FUNCTION_BLOCK "IMAC_MOTOR1"
TITLE = MOTOR 1
//--------------------------------------------------------------------------------
//SIEMENS AG     I&S IP PEP SN                       PSP-Element: D-09300081-E-E5
//--------------------------------------------------------------------------------
//History
//=======
//Date      Version  Description                        Author
//1997/06/09   0.6   Basic Edition                      Salge
//2004/06/02   1.0   Converted to S7                    Kahle
//2004/11/29   1.1   Anypointer adjusted                Edelmann
//2004/12/07   1.2   Interface adapted                  Edelmann
//
//--------------------------------------------------------------------------------
//PLC:   >= S7-300
//--------------------------------------------------------------------------------
//Specification:   Refer "TECHFUNK.DOC"
//--------------------------------------------------------------------------------
//
//--------------------------------------------------------------------------------
//Called FC: FC90 "DELAYTIMER"
//           SFC20 "BLKMOV"
//--------------------------------------------------------------------------------
//
//--------------------------------------------------------------------------------
//Note:
//--------------------------------------------------------------------------------
// KNOW_HOW_PROTECT
AUTHOR : Sa_Ka
FAMILY : IMAC
NAME : Motor1
VERSION : 1.2


VAR_INPUT
  OBJ : INT ;	//current used object
  RMOT : BOOL ;	//mode remote (=1) is activated
  RUN : BOOL ;	//Feedback Motor is running
  FAUL : BOOL ;	//Feedback Motor fault
  BLKO : BOOL ;	//Blackout indication
  ACOM : WORD ;	//Automatic commands
  PCONF : STRUCT
   LastRecord : INT  := 100;
   Pointer1stRecord : STRUCT
    S7ID : BYTE  := B#16#10;	//ANY pointer: ID S7
    Typ : BYTE  := B#16#2;	//ANY pointer: data typ =02 BYTE =04 WORD =05 INT =06 DWORD =07 DINT =08 REAL
    RepeatFactor : INT  := 104;	//ANY pointer: repeat factor
    DBNo : INT  := 80;	//ANY pointer: DB number, zero if no DB
    MemoryArea : BYTE  := B#16#84;	//ANY pointer: Memory area =81 IN =82 OUT =83 M =84 DB =85 DI =86 L
    DWHigh : BYTE ;	//ANY pointer: DW highest byte
    DWX : INT ;	//ANY pointer: DW low / bit (address = byte *8 + bit)
   END_STRUCT ;
  END_STRUCT ;
END_VAR
VAR_OUTPUT
  MSTA : BOOL ;	//Command Start Motor
  MSTO : BOOL ;	//Command Stop Motor
  ASTAT : WORD ;	//Status as feedback for the automatic
//******************** CODE SECTION ********
  OSSTAT : WORD ;	//Status for OS
  OSALARM : WORD ;	//Alarms for OS
END_VAR
VAR_IN_OUT
  OSCOM : WORD ;
END_VAR
VAR
  Motor1 : STRUCT
   System : WORD ;
   CmdOS : WORD ;
   MirrorCmdOS : WORD ;
   Test : WORD ;
   AlarmOS : WORD ;
   StatusOS : WORD ;
   SysStatusOS : WORD ;
   Status1 : WORD ;
   Status2 : WORD ;
   InputEdges : WORD ;
   AutoEdges : WORD ;
   DataTimeCmd : STRUCT
    StartTime : DINT ;
    StartEdge : BOOL ;
   END_STRUCT ;
   DataTimeBlackout : STRUCT
    StartTime : DINT ;
    StartEdge : BOOL ;
   END_STRUCT ;
   DataTimeExtFault : STRUCT
    StartTime : DINT ;
    StartEdge : BOOL ;
   END_STRUCT ;
   DataTimeFeedback : STRUCT
    StartTime : DINT ;
    StartEdge : BOOL ;
   END_STRUCT ;
   DataTimeStrtActFault : STRUCT
    StartTime : DINT ;
    StartEdge : BOOL ;
   END_STRUCT ;
   DataTimeAutoAl : STRUCT
    StartTime : DINT ;
    StartEdge : BOOL ;
   END_STRUCT ;
   DataTimeRestart : STRUCT
    StartTime : DINT ;
    StartEdge : BOOL ;
   END_STRUCT ;
   DataTimeStpActFault : STRUCT
    StartTime : DINT ;
    StartEdge : BOOL ;
   END_STRUCT ;
   PCONF : STRUCT
    Modeswitches : STRUCT
     DlyAFaultStop : BOOL ;	//    Modeswitch Delayed Auto Fault with Stop
     sw01 : BOOL ;	//
     ExtFaultNC : BOOL ;	//    Modeswitch External fault NC
     sw03 : BOOL ;	//
     sw04 : BOOL ;	//
     sw05 : BOOL ;	//
     sw06 : BOOL ;	//
     sw07 : BOOL ;	//
     ConstOutput : BOOL ;	//    Modeswitch Constant Output
     ExtraAutomode : BOOL ;	//    Extra Automode
     NoActAFeedbackA : BOOL ;	//    Modeswitch No action and feedback alarm
     StopIfA : BOOL ;	//    Modeswitch Stop if alarm
     RestrtAftBlack : BOOL ;	//    Modeswitch Restart after Blackout
     RstAStartStop : BOOL ;	//    Modeswitch Reset Alarm with Start /Stop
     CmdTdly : BOOL ;	//    Modeswitch Command time delay
     LockBlockCmd : BOOL ;	//    Modeswitch Lock blocksCommands
    END_STRUCT ;
    DlyTCmd : TIME ;	// Setpoint command time delay
    DlyTBlackout : TIME ;	// Setpoint blackout time delay
    DlyTExtFault : TIME ;	// Setpoint external fault delay
    DlyTFeedback : TIME ;	// Setpoint feedback fault delay
    DlyTStrtActFault : TIME ;	//Setpoint start action delay
    DlyTAutoAl : TIME ;	// Setpoint auto alarm delay
    DlyTRestart : TIME ;	// Setpoint restart after blackout delay
    DlyTStpActFault : TIME ;	// Setpoint stop action fault
   END_STRUCT ;
  END_STRUCT ;
  siFailRR : INT ;	//Failure blockmove read record
  siFailWR : INT ;	//Failure blockmove write record
END_VAR
VAR_TEMP
  tb200_0 : BOOL ;	//
  tbCmdOSManual : BOOL ;	//    Command Manual
  tbCmdOSAuto : BOOL ;	//    Command Auto
  tb200_3 : BOOL ;	//
  tb200_4 : BOOL ;	//
  tb200_5 : BOOL ;	//
  tb200_6 : BOOL ;	//
  tb200_7 : BOOL ;	//
  tbCmdOSStart : BOOL ;	//    Command Start OS pulse
  tbCmdOSStop : BOOL ;	//    Command Stop OS pulse
  tb201_2 : BOOL ;	//
  tb201_3 : BOOL ;	//
  tb201_4 : BOOL ;	//
  tb201_5 : BOOL ;	//
  tb201_6 : BOOL ;	//
  tbCmdOSReset : BOOL ;	//    Command Reset OS pulse
  tbAutoBlackStart : BOOL ;	//    Blackoutstart from Auto
  tbAutoStbyCtrl : BOOL ;	//    Standbycontrol active
  tb202_2 : BOOL ;	//
  tb202_3 : BOOL ;	//
  tb202_4 : BOOL ;	//
  tb202_5 : BOOL ;	//
  tb202_6 : BOOL ;	//
  tbDataReq : BOOL ;	//    Fetch Data requiered
  tbAutoStart : BOOL ;	//
  tbAutoStop : BOOL ;	//
  tbAutoFail : BOOL ;	//    Auto failure input
  tbCmdLock : BOOL ;	//    Command Lock
  tbCmdEmergOff : BOOL ;	//    Command Emergency Off
  tb203_5 : BOOL ;	//
  tb203_6 : BOOL ;	//
  tb203_7 : BOOL ;	//
  tb204_0 : BOOL ;	//
  tb204_1 : BOOL ;	//
  tb204_2 : BOOL ;	//
  tb204_3 : BOOL ;	//
  tb204_4 : BOOL ;	//
  tb204_5 : BOOL ;	//
  tb204_6 : BOOL ;	//
  tb204_7 : BOOL ;	//
  tbCmdAutoStart : BOOL ;	//    Command Start Auto Pulse
  tbCmdAutoStop : BOOL ;	//    Command Stop Auto Pulse
  tbCmdAutoFail : BOOL ;	//    Auto failure input pulse
  tb205_3 : BOOL ;	//
  tb205_4 : BOOL ;	//
  tb205_5 : BOOL ;	//
  tb205_6 : BOOL ;	//
  tb205_7 : BOOL ;	//
  tbRemote : BOOL ;	//    Remote (=1)/ Local
  tbRunning : BOOL ;	//    Running (=1)/ Stopped
  tbFault : BOOL ;	//    Fault
  tbBlackout : BOOL ;	//    Blackout
  tb206_4 : BOOL ;	//
  tb206_5 : BOOL ;	//
  tb206_6 : BOOL ;	//
  tb206_7 : BOOL ;	//
  tb207_0 : BOOL ;	//
  tb207_1 : BOOL ;	//
  tb207_2 : BOOL ;	//
  tb207_3 : BOOL ;	//
  tb207_4 : BOOL ;	//
  tb207_5 : BOOL ;	//
  tb207_6 : BOOL ;	//
  tb207_7 : BOOL ;	//
  tb208_0 : BOOL ;	//
  tb208_1 : BOOL ;	//
  tb208_2 : BOOL ;	//
  tb208_3 : BOOL ;	//
  tb208_4 : BOOL ;	//
  tb208_5 : BOOL ;	//
  tb208_6 : BOOL ;	//
  tbSendData : BOOL ;	//    Send Data
  tbStateRun : BOOL ;	//    State Running
  tbStateLocal : BOOL ;	//    State Local
  tbStateManual : BOOL ;	//    State Manual
  tbStateAuto : BOOL ;	//    State Auto
  tbStateFault : BOOL ;	//    State Fault
  tbStateBlackout : BOOL ;	//    State Blackout
  tbStarting : BOOL ;	//    Starting
  tbReStarting : BOOL ;	//    ReStarting
  tb210_0 : BOOL ;
  tb210_1 : BOOL ;
  tb210_2 : BOOL ;
  tb210_3 : BOOL ;
  tb210_4 : BOOL ;
  tb210_5 : BOOL ;
  tb210_6 : BOOL ;
  tb210_7 : BOOL ;
  tb211_0 : BOOL ;
  tb211_1 : BOOL ;
  tb211_2 : BOOL ;
  tb211_3 : BOOL ;
  tb211_4 : BOOL ;
  tb211_5 : BOOL ;
  tb211_6 : BOOL ;
  tb211_7 : BOOL ;
  tb212_0 : BOOL ;
  tb212_1 : BOOL ;
  tb212_2 : BOOL ;
  tb212_3 : BOOL ;
  tb212_4 : BOOL ;
  tb212_5 : BOOL ;
  tb212_6 : BOOL ;
  tb212_7 : BOOL ;
  tb213_0 : BOOL ;
  tb213_1 : BOOL ;
  tb213_2 : BOOL ;
  tb213_3 : BOOL ;
  tb213_4 : BOOL ;
  tb213_5 : BOOL ;
  tb213_6 : BOOL ;
  tb213_7 : BOOL ;
  tbNonFeedbackTact : BOOL ;	//    Non Feedback Timer active
  tbNonFeedbackA : BOOL ;	//    Non Feedback Alarm
  tbStartTact : BOOL ;	//    Start Timer active
  tbActionA : BOOL ;	//    Action Alarm
  tbAutoTact : BOOL ;	//    Auto Timer active
  tbAutoA : BOOL ;	//    Auto Alarm
  tbRunBeforeBlack : BOOL ;	//    Running before blackout
  tbBlackoutStartTact : BOOL ;	//    Blackout start timer active
  tbStart : BOOL ;	//    Start
  tbStop : BOOL ;	//    Stop
  tbLocal : BOOL ;	//    Local
  tbManual : BOOL ;	//    Manual
  tbAuto : BOOL ;	//    Auto
  tbCmdTact : BOOL ;	//    Command Timer activ
  tbFaultTact : BOOL ;	//    Fault timer active
  tbExtFaultA : BOOL ;	//    Fault input alarm / external fault alarm
  tbMSTA : BOOL ;	//    Output MSTA
  tbMSTO : BOOL ;	//    Output MSTO
  tb216_2 : BOOL ;	//
  tb216_3 : BOOL ;	//
  tb216_4 : BOOL ;	//
  tb216_5 : BOOL ;	//
  tb216_6 : BOOL ;	//
  tb216_7 : BOOL ;	//
  tbDlyStop : BOOL ;	//    Delayed stop
  tbDlyStart : BOOL ;	//    Delayed start
  tbStopTact : BOOL ;	//    Stop Timer active
  tb217_3 : BOOL ;	//
  tb217_4 : BOOL ;	//
  tb217_5 : BOOL ;	//
  tb217_6 : BOOL ;	//
  tb217_7 : BOOL ;	//
  tbLtRpulse : BOOL ;	//    Local to remote pulse
  tb218_1 : BOOL ;	//
  tb218_2 : BOOL ;	//
  tb218_3 : BOOL ;	//
  tb218_4 : BOOL ;	//
  tb218_5 : BOOL ;	//
  tb218_6 : BOOL ;	//
  tb218_7 : BOOL ;	//
  tb219_0 : BOOL ;	//
  tb219_1 : BOOL ;	//
  tb219_2 : BOOL ;	//
  tb219_3 : BOOL ;	//
  tb219_4 : BOOL ;	//
  tb219_5 : BOOL ;	//
  tb219_6 : BOOL ;	//
  tb219_7 : BOOL ;	//
  tbCmdTexceed : BOOL ;	//Commnd delay time exceeded
  tbStartTexceed : BOOL ;	//Start delay time exceeded
  tbExtFTexceed : BOOL ;	//External fault delay time exceeded
  tbFeedbackTexceed : BOOL ;	//Feedback delay time exceeded
  tbAutoTexceed : BOOL ;	//Auto delay time exceeded
  tbBOStartTexceed : BOOL ;	//Blackout start delay time exceeded
  tb250_6 : BOOL ;
  tbStopTexceed : BOOL ;	//Stop delay time exceeded
  tbStartPulse : BOOL ;
  tbStopPulse : BOOL ;
  P_currentRecord : ANY ;	//ANY pointer of the current record
END_VAR
BEGIN
NETWORK
TITLE =Calculation of current ANY pointer for reading /writing record
// ANY-pointer of current record
      L     #PCONF.Pointer1stRecord.S7ID;
      T     LB    22;
      L     #PCONF.Pointer1stRecord.Typ;
      T     LB    23;
      L     #PCONF.Pointer1stRecord.RepeatFactor;
      T     LW    24;
      L     #PCONF.Pointer1stRecord.DBNo;
      T     LW    26;
      L     #PCONF.Pointer1stRecord.MemoryArea;
      T     LB    28;
      L     #PCONF.Pointer1stRecord.DWHigh;
      T     LB    29;
      L     #PCONF.Pointer1stRecord.DWX;
      T     LW    30;

      L     #OBJ; //Check whether Obj within the range
      L     #PCONF.LastRecord;
      >I    ;
      SPB   cRcd;
      L     #OBJ;
      L     1;
      <I    ;
      SPB   cRcd;
      L     #OBJ;
cRcd: +     -1;
      L     #PCONF.Pointer1stRecord.RepeatFactor;
      *I    ;
      SLD   3; //DBW + DBX address of the current record
      L     LD    28;
      OD    ;
      T     LD    28; //DBWX part of ANY pointer "P_currentRecord"

NETWORK
TITLE =Read record

      CALL "BLKMOV" (
           SRCBLK                   := #P_currentRecord,
           RET_VAL                  := #siFailRR,
           DSTBLK                   := #Motor1);


NETWORK
TITLE =Read Record

      L     #OSCOM; // Commands from OS
      T     LW     0;
      L     #Motor1.Status1; // Status stored
      T     LW    14;
      L     #Motor1.Status2; // Status stored
      T     LW    16;

      L     0; //Reset scratch  flags
      T     LW     6;
      T     LW    20;
      NOP   0;


NETWORK
TITLE =Formaloperanden Inputs
//// NW 3 Formaloperanden einlesen
//
//
      U     #RMOT;
      =     #tbRemote; // Remote/Local
      U     #RUN;
      =     #tbRunning; // Running/Stopped

      U     #Motor1.PCONF.Modeswitches.ExtFaultNC; //Modswitch External Fault NC
      SPB   NC; //jump Normal Closed Input
      U     #FAUL;
      =     #tbFault; // Fault
      SPA   GO;
NC:   UN    #FAUL;
      =     #tbFault; // Fault

GO:   L     #ACOM;
      T     LW     2; // Command From Automatic
      U     #BLKO;
      =     #tbBlackout; //Blackout

// ----Evaluate Pulsflags from Auto Commands----
      L     #Motor1.AutoEdges; //Stored Auto Command last cycle
      INVI  ; //Singlecomplement
      L     LW     2; //Command From Automatic
      T     #Motor1.AutoEdges; //
      UW    ;
      T     LW     4; // Command  Pulseflags

// ----Evaluate Pulsflags from Inputs----
      L     #Motor1.InputEdges; //Stored Inputs last cycle
      INVI  ; //Singlecomplement
      L     LB     6; //Inputs
      T     #Motor1.InputEdges; //
      UW    ;
      T     LB    18; // Inputs Pulseflags
      NOP   0;


NETWORK
TITLE =Local-Manual- Auto
//// NW 4  Local-Manual- Auto
      UN    #tbRemote; // Not Remote
      =     #tbLocal; // LOCAL
      R     #tbManual; // MANUAL!
      R     #tbAuto; // AUTO!
      R     #tbDlyStart; // DELAYDED START!
      R     #tbDlyStop; // DELAYDED STOP!
      R     #tbCmdTact; // reset COMMAND TIMER ACTIV
      R     #tbStart; // START!
      R     #tbStop; // STOP!
      R     #tbRunBeforeBlack; // RUNNING BEFORE BLACKOUT
      R     #tbNonFeedbackTact; // reset Non Feedback Timer
      R     #tbStartTact; // reset Start Timer
      R     #tbStopTact; // reset Stop Timer
      R     #tbAutoTact; // reset Auto Timer
      SPB   NE4;
      U     #Motor1.PCONF.Modeswitches.ExtraAutomode; // extra Automode ?
      SPB   MODE;
      S     #tbManual; //MANUAL!
      S     #tbAuto; // AUTO!
      SPA   NE4;
MODE: U     #tbCmdOSManual; //Command Manual
      S     #tbManual; //MANUAL!
      R     #tbAuto; // AUTO!
      U     #tbCmdOSAuto; //Command Auto
      S     #tbAuto; // AUTO!
      R     #tbManual; // MANUAL!
      UN    #tbAuto; // AUTO!
      UN    #tbManual; // MANUAL!
      S     #tbManual; // MANUAL!
NE4:  NOP   0;

NETWORK
TITLE =Commands
//-------SET Start Command----------
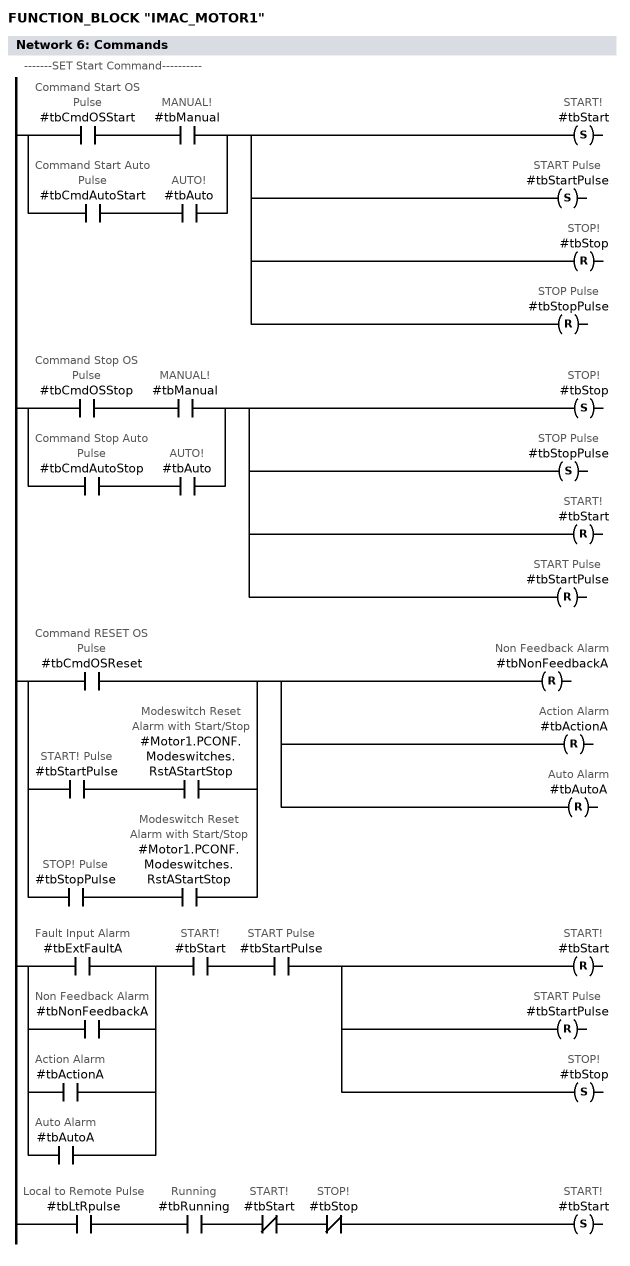
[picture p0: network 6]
      O(    ;
      U     #tbCmdOSStart; //Command Start OS Pulse
      U     #tbManual; // MANUAL!
      )     ;
      O(    ;
      U     #tbCmdAutoStart; //Command Start Auto Pulse
      U     #tbAuto; // AUTO!
      )     ;
      S     #tbStart; // START!
      S     #tbStartPulse; // START Pulse
      R     #tbStop; // STOP!
      R     #tbStopPulse; // STOP Pulse

//-------SET Stop Command----------
      O(    ;
      U     #tbCmdOSStop; //Command Stop OS Pulse
      U     #tbManual; // MANUAL!
      )     ;
      O(    ;
      U     #tbCmdAutoStop; //Command Stop Auto Pulse
      U     #tbAuto; // AUTO!
      )     ;
      S     #tbStop; // STOP!
      S     #tbStopPulse; // STOP Pulse
      R     #tbStart; // START!
      R     #tbStartPulse; // START Pulse

//-------Reset Alarms----------
      O     #tbCmdOSReset; //Command RESET OS Pulse
      O(    ;
      U     #tbStartPulse; // START! Pulse
      U     #Motor1.PCONF.Modeswitches.RstAStartStop; // Modeswitch Reset Alarm with Start/Stop
      )     ;
      O(    ;
      U     #tbStopPulse; // STOP! Pulse
      U     #Motor1.PCONF.Modeswitches.RstAStartStop; // Modeswitch Reset Alarm with Start/Stop
      )     ;
      R     #tbNonFeedbackA; // Non Feedback Alarm
      R     #tbActionA; // Action Alarm
      R     #tbAutoA; // Auto Alarm

//-------Reset START ! if Failure----------
      O     #tbExtFaultA; // Fault Input Alarm
      O     #tbNonFeedbackA; // Non Feedback Alarm
      O     #tbActionA; // Action Alarm
      O     #tbAutoA; // Auto Alarm
      U     #tbStart; // START!
      U     #tbStartPulse; // START Pulse
      R     #tbStart; // START!
      R     #tbStartPulse; // START Pulse
      S     #tbStop; // STOP!

//-------Local Remote change ----------
      U     #tbLtRpulse; // Local to Remote Pulse
      U     #tbRunning; // Running
      UN    #tbStart; // START!
      UN    #tbStop; // STOP!
      S     #tbStart; // START!
      NOP   0;



NETWORK
TITLE =Command Time Delay

      UN    #Motor1.PCONF.Modeswitches.CmdTdly; // no Modeswitch Command time delay ?
      SPB   NE6;
      U     #tbCmdTact; // COMMAND TIMER ACTIV
      U     #tbStartPulse; // START! Pulse
      R     #tbStartPulse; // reset START! Pulse
      R     #tbStart; // reset START!
      S     #tbDlyStart; // DELAYDED START!
      R     #tbDlyStop; // DELAYDED STOP!

      U     #tbCmdTact; // COMMAND TIMER ACTIV
      U     #tbStopPulse; // STOP! Pulse
      R     #tbStopPulse; // reset STOP! Pulse
      R     #tbStop; // reset STOP!
      S     #tbDlyStop; // DELAYDED STOP!
      R     #tbDlyStart; // DELAYDED START!

      O     #tbStartPulse; // START! Pulse
      O     #tbStopPulse; // STOP! Pulse
      S     #tbCmdTact; // set COMMAND TIMER ACTIV +++Input FB97

      CALL "IMAC_DELAYTIMER" (
           XSTART                   := #tbCmdTact,
           XTIME                    := #Motor1.PCONF.DlyTCmd,
           YON                      := #tbCmdTexceed,
           MEM                      := #Motor1.DataTimeCmd);

      U     #tbCmdTexceed; // Command Time is over pulse
      U     #tbDlyStart; // DELAYDED START!
      S     #tbStart; // START!
      S     #tbStartPulse; // START! Pulse
      R     #tbDlyStart; // DELAYDED START!

      U     #tbCmdTexceed; // Command Time is over pulse
      U     #tbDlyStop; // DELAYDED STOP!
      S     #tbStop; // STOP!
      S     #tbStopPulse; // STOP! Pulse
      R     #tbDlyStop; // DELAYDED STOP!

NE6:  NOP   0;
NETWORK
TITLE =Restart after Blackout
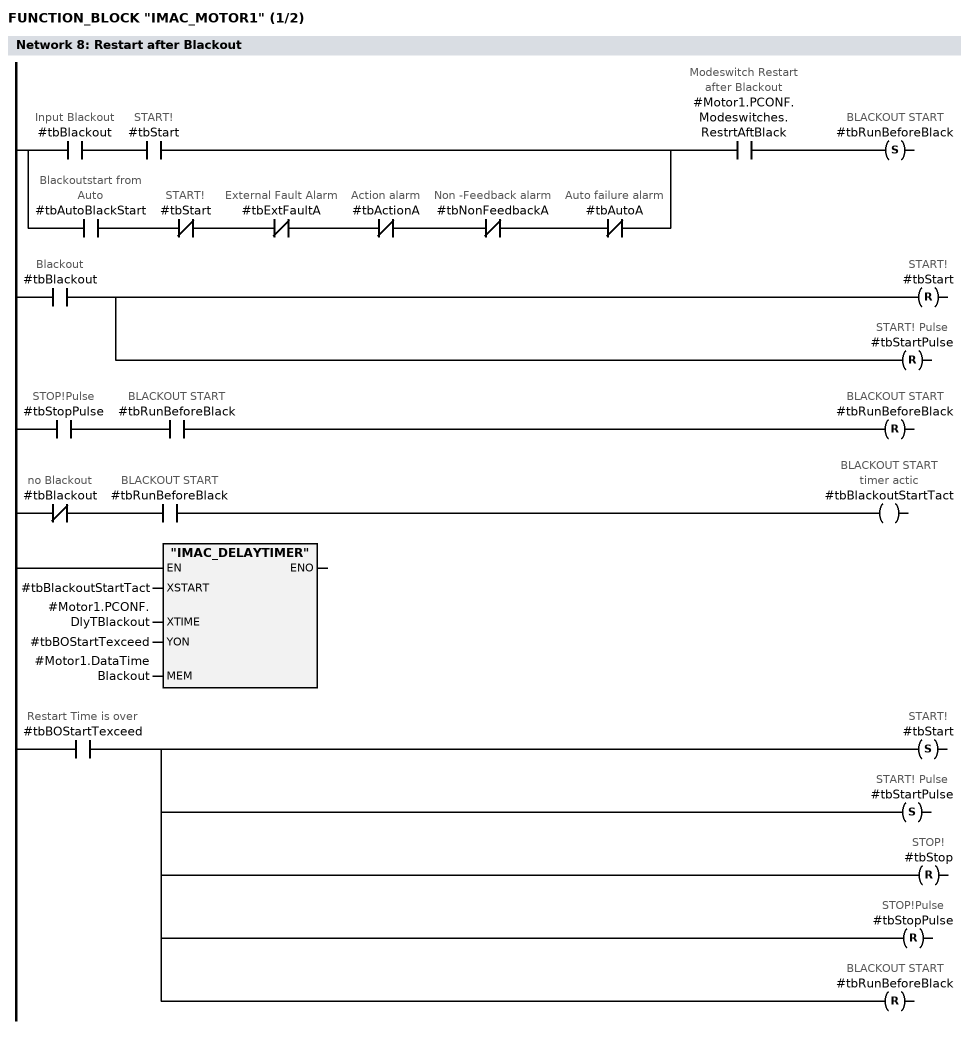
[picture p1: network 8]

      O(    ;
      U     #tbBlackout; // Input Blackout
      U     #tbStart; // START!
      )     ;
      O(    ;
      U     #tbAutoBlackStart; // Blackoutstart from  Auto
      UN    #tbStart; // START!
      UN    #tbExtFaultA; // External Fault Alarm
      UN    #tbActionA; // Action alarm
      UN    #tbNonFeedbackA; // Non -Feedback alarm
      UN    #tbAutoA; // Auto failure alarm
      )     ;
      U     #Motor1.PCONF.Modeswitches.RestrtAftBlack; // Modeswitch Restart after Blackout
      S     #tbRunBeforeBlack; // BLACKOUT START

      U     #tbBlackout; // Blackout
      R     #tbStart; // START!
      R     #tbStartPulse; // START! Pulse

      U     #tbStopPulse; // STOP!Pulse
      U     #tbRunBeforeBlack; // BLACKOUT START
      R     #tbRunBeforeBlack; // BLACKOUT START

      UN    #tbBlackout; //  no Blackout
      U     #tbRunBeforeBlack; // BLACKOUT START
      =     #tbBlackoutStartTact; // BLACKOUT START timer actic
      CALL "IMAC_DELAYTIMER" (
           XSTART                   := #tbBlackoutStartTact,
           XTIME                    := #Motor1.PCONF.DlyTBlackout,
           YON                      := #tbBOStartTexceed,
           MEM                      := #Motor1.DataTimeBlackout);

      U     #tbBOStartTexceed; // Restart Time is over
      S     #tbStart; // START!
      S     #tbStartPulse; // START! Pulse
      R     #tbStop; // STOP!
      R     #tbStopPulse; // STOP!Pulse
      R     #tbRunBeforeBlack; // BLACKOUT START
      NOP   0;
NETWORK
TITLE =Action Alarm
//------- Start Action-------------
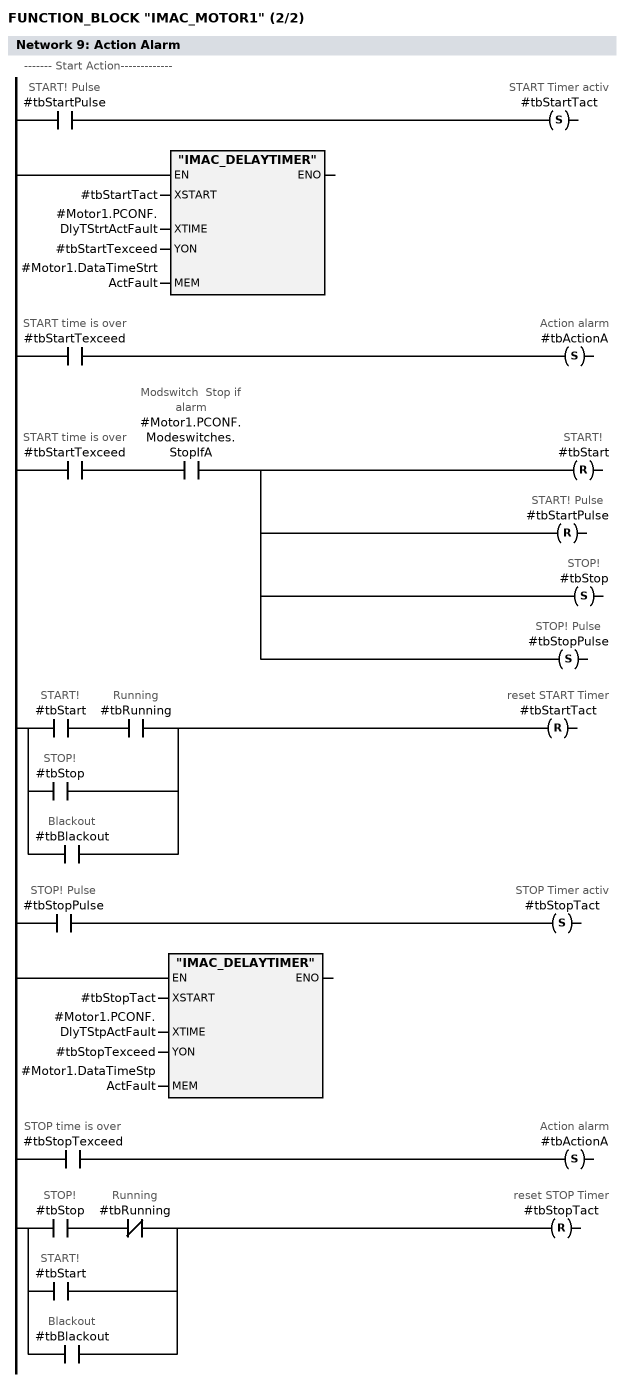
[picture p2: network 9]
      U     #tbStartPulse; // START! Pulse
      S     #tbStartTact; // START Timer activ
      CALL "IMAC_DELAYTIMER" (
           XSTART                   := #tbStartTact,
           XTIME                    := #Motor1.PCONF.DlyTStrtActFault,
           YON                      := #tbStartTexceed,
           MEM                      := #Motor1.DataTimeStrtActFault);

      U     #tbStartTexceed; // START time is over
      S     #tbActionA; // Action alarm
      U     #tbStartTexceed; // START time is over
      U     #Motor1.PCONF.Modeswitches.StopIfA; // Modswitch  Stop if alarm
      R     #tbStart; // START!
      R     #tbStartPulse; // START! Pulse
      S     #tbStop; // STOP!
      S     #tbStopPulse; // STOP! Pulse

      U     #tbStart; // START!
      U     #tbRunning; // Running
      O     #tbStop; // STOP!
      O     #tbBlackout; // Blackout
      R     #tbStartTact; // reset START Timer

//------- Stop Action-------------
      U     #tbStopPulse; // STOP! Pulse
      S     #tbStopTact; // STOP Timer activ
      CALL "IMAC_DELAYTIMER" (
           XSTART                   := #tbStopTact,
           XTIME                    := #Motor1.PCONF.DlyTStpActFault,
           YON                      := #tbStopTexceed,
           MEM                      := #Motor1.DataTimeStpActFault);

      U     #tbStopTexceed; // STOP time is over
      S     #tbActionA; // Action alarm

      U     #tbStop; // STOP!
      UN    #tbRunning; // Running
      O     #tbStart; // START!
      O     #tbBlackout; // Blackout
      R     #tbStopTact; // reset STOP Timer
      NOP   0;
NETWORK
TITLE =External Fault Alarm

      O     #tbAuto; // AUTO!
      O     #tbManual; // MANUAL!
      SPB   RMOT;
      U     #tbFault; // External Fault
      =     #tbExtFaultA; // External Fault Alarm
      SPA   NE8;
RMOT: U     #tbFault; // External Fault
      UN    #tbExtFaultA; // External Fault Alarm
      UN    #tbBlackout; // Blackout
      =     #tbFaultTact; // Fault timer activ
      CALL "IMAC_DELAYTIMER" (
           XSTART                   := #tbFaultTact,
           XTIME                    := #Motor1.PCONF.DlyTExtFault,
           YON                      := #tbExtFTexceed,
           MEM                      := #Motor1.DataTimeExtFault);

      U     #tbExtFTexceed; // Fault time over
      S     #tbExtFaultA; // External Fault Alarm
      R     #tbStart; // START!
      R     #tbStartPulse; // START! Pulse
      S     #tbStop; // STOP!
      S     #tbStopPulse; // STOP! Pulse

      UN    #tbFault; // External Fault
      R     #tbExtFaultA; // Fault Input Alarm

NE8:  NOP   0;
NETWORK
TITLE =Non-Feedback alarm

      U     #Motor1.PCONF.Modeswitches.NoActAFeedbackA; // Modeswitch No Action and Feedback alarm
      SPB   NE9;
      O(    ;
      U     #tbStart; // START!
      UN    #tbRunning; // not Running
      )     ;
      O(    ;
      U     #tbStop; // STOP!
      U     #tbRunning; // Running
      )     ;
      UN    #tbNonFeedbackA; // Non -Feedback alarm
      UN    #tbStartTact; // no Start Timer activ
      UN    #tbStopTact; // no Stop Timer activ
      UN    #tbActionA; // no Action alarm
      UN    #tbFaultTact; // no Fault timer activ
      UN    #tbExtFaultA; // no External Fault Alarm
      UN    #tbBlackout; // no Blackout
      =     #tbNonFeedbackTact; // Non -Feedback Timer activ
      CALL "IMAC_DELAYTIMER" (
           XSTART                   := #tbNonFeedbackTact,
           XTIME                    := #Motor1.PCONF.DlyTFeedback,
           YON                      := #tbFeedbackTexceed,
           MEM                      := #Motor1.DataTimeFeedback);

      U     #tbFeedbackTexceed; // Non -Feedback time is over
      S     #tbNonFeedbackA; // Non -Feedback alarm
      U     #tbFeedbackTexceed; // Non -Feedback time is over
      U     #Motor1.PCONF.Modeswitches.StopIfA; // Modswitch  Stop iif alarm
      U     #tbStart; // START!
      R     #tbStart; // START!
      R     #tbStartPulse; // START! Pulse
      S     #tbStop; // STOP!
      S     #tbStopPulse; // STOP! Pulse

NE9:  NOP   0;
NETWORK
TITLE =Auto Failure

      UN    #tbAuto; // not in AUTO! Mode
      SPB   NE10;
      U     #tbCmdAutoFail; // Auto failure Input pulse
      S     #tbAutoTact; // Auto failure Timer activ
      UN    #tbAutoFail; // Auto failure Input
      R     #tbAutoTact; // Auto failure Timer activ
      CALL "IMAC_DELAYTIMER" (
           XSTART                   := #tbAutoTact,
           XTIME                    := #Motor1.PCONF.DlyTAutoAl,
           YON                      := #tbAutoTexceed,
           MEM                      := #Motor1.DataTimeAutoAl);

      U     #tbAutoTexceed; // Auto failure time is over
      S     #tbAutoA; // Auto failure alarm
      U     #tbAutoTexceed; // Auto failure time is over
      U     #Motor1.PCONF.Modeswitches.DlyAFaultStop; // Modeswitch Delayded AutoFault with Stop
      R     #tbStart; // START!
      R     #tbStartPulse; // START! Pulse
      S     #tbStop; // STOP!
      S     #tbStopPulse; // STOP! Pulse

NE10: NOP   0;
NETWORK
TITLE =Automatic States
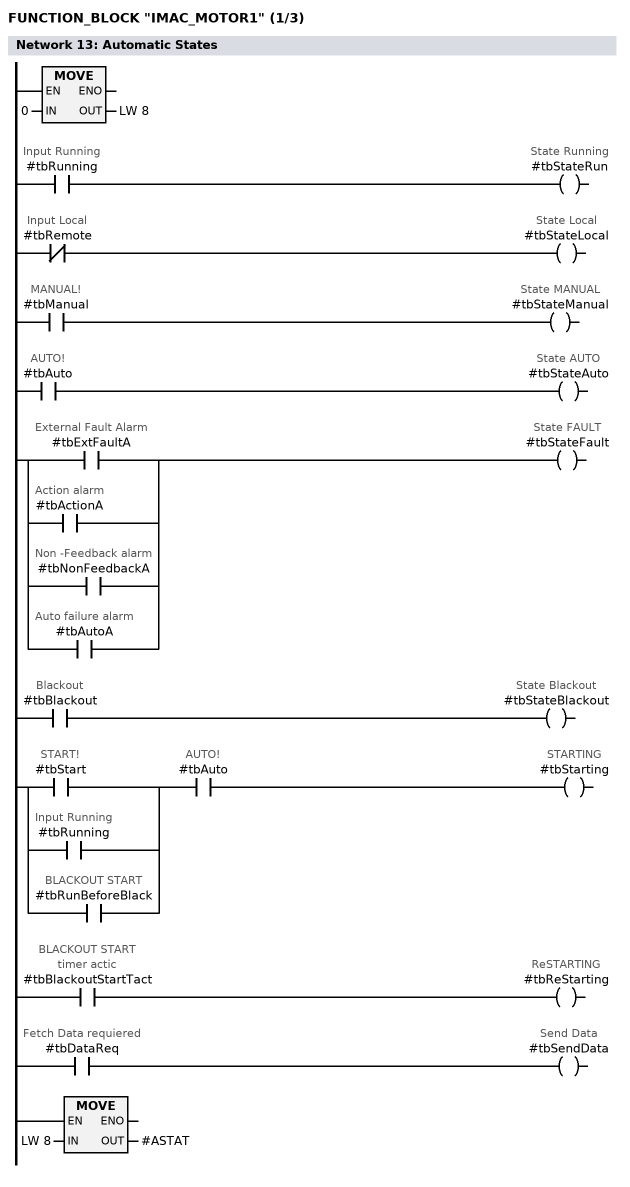
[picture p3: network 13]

      L     0;
      T     LW     8;
      U     #tbRunning; // Input Running
      =     #tbStateRun; // State Running
      UN    #tbRemote; // Input Local
      =     #tbStateLocal; // State Local
      U     #tbManual; // MANUAL!
      =     #tbStateManual; // State MANUAL
      U     #tbAuto; // AUTO!
      =     #tbStateAuto; // State AUTO
      O     #tbExtFaultA; // External Fault Alarm
      O     #tbActionA; // Action alarm
      O     #tbNonFeedbackA; // Non -Feedback alarm
      O     #tbAutoA; // Auto failure alarm
      =     #tbStateFault; // State FAULT
      U     #tbBlackout; // Blackout
      =     #tbStateBlackout; // State Blackout
      O     #tbStart; // START!
      O     #tbRunning; // Input Running
      O     #tbRunBeforeBlack; // BLACKOUT START
      U     #tbAuto; // AUTO!
      =     #tbStarting; // STARTING
      U     #tbBlackoutStartTact; // BLACKOUT START timer actic
      =     #tbReStarting; // ReSTARTING
      U     #tbDataReq; // Fetch Data requiered
      =     #tbSendData; // Send Data
      L     LW     8;
      T     #ASTAT;
      NOP   0;
NETWORK
TITLE =Lock/ Emergency Off
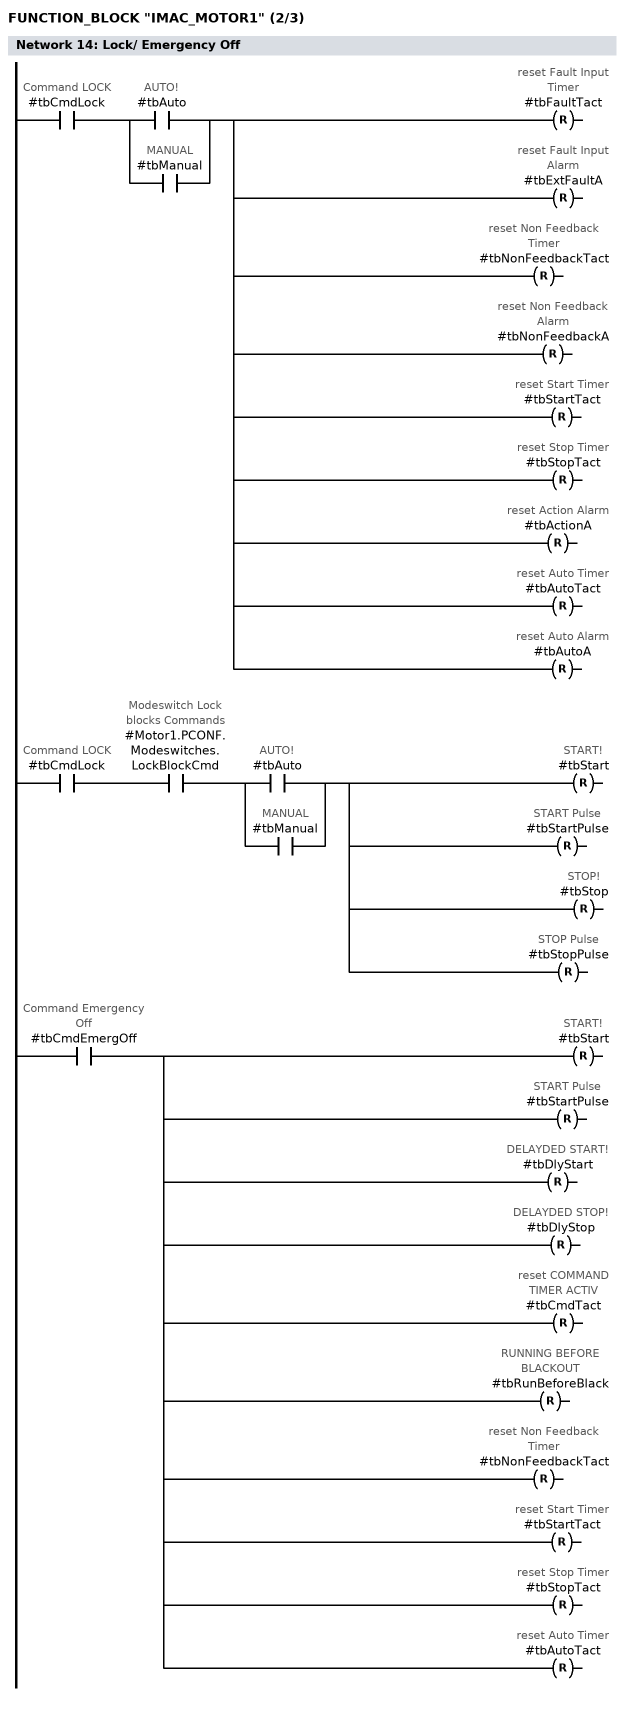
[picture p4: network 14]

      U     #tbCmdLock; //Command LOCK
      U(    ;
      O     #tbAuto; // AUTO!
      O     #tbManual; // MANUAL
      )     ;
      R     #tbFaultTact; // reset Fault Input Timer
      R     #tbExtFaultA; // reset Fault Input Alarm
      R     #tbNonFeedbackTact; // reset Non Feedback Timer
      R     #tbNonFeedbackA; // reset Non Feedback Alarm
      R     #tbStartTact; // reset Start Timer
      R     #tbStopTact; // reset Stop Timer
      R     #tbActionA; // reset Action Alarm
      R     #tbAutoTact; // reset Auto Timer
      R     #tbAutoA; // reset Auto Alarm

      U     #tbCmdLock; //Command LOCK
      U     #Motor1.PCONF.Modeswitches.LockBlockCmd; //Modeswitch Lock blocks Commands
      U(    ;
      O     #tbAuto; // AUTO!
      O     #tbManual; // MANUAL
      )     ;
      R     #tbStart; // START!
      R     #tbStartPulse; // START Pulse
      R     #tbStop; // STOP!
      R     #tbStopPulse; // STOP Pulse

//----Emergency Off
      U     #tbCmdEmergOff; //Command Emergency Off
      R     #tbStart; // START!
      R     #tbStartPulse; // START Pulse

      R     #tbDlyStart; // DELAYDED START!
      R     #tbDlyStop; // DELAYDED STOP!
      R     #tbCmdTact; // reset COMMAND TIMER ACTIV
      R     #tbRunBeforeBlack; // RUNNING BEFORE BLACKOUT
      R     #tbNonFeedbackTact; // reset Non Feedback Timer
      R     #tbStartTact; // reset Start Timer
      R     #tbStopTact; // reset Stop Timer
      R     #tbAutoTact; // reset Auto Timer
      NOP   0;
NETWORK
TITLE =Output
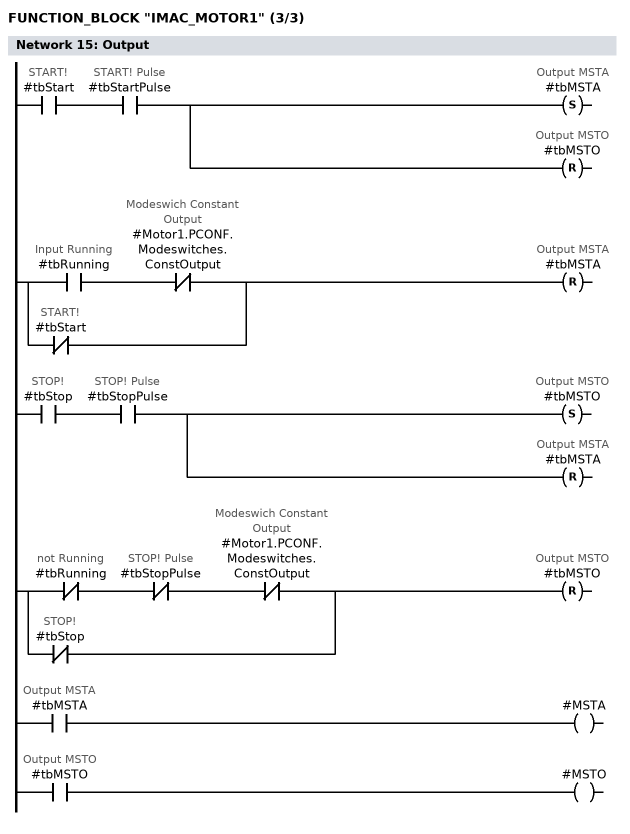
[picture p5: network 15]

      U     #tbStart; // START!
      U     #tbStartPulse; // START! Pulse
      S     #tbMSTA; // Output MSTA
      R     #tbMSTO; // Output MSTO
      U     #tbRunning; // Input Running
      UN    #Motor1.PCONF.Modeswitches.ConstOutput; // Modeswich Constant Output
      ON    #tbStart; // START!
      R     #tbMSTA; // Output MSTA

      U     #tbStop; // STOP!
      U     #tbStopPulse; // STOP! Pulse
      S     #tbMSTO; // Output MSTO
      R     #tbMSTA; // Output MSTA

      UN    #tbRunning; // not Running
      UN    #tbStopPulse; // STOP! Pulse
      UN    #Motor1.PCONF.Modeswitches.ConstOutput; // Modeswich Constant Output
      ON    #tbStop; // STOP!
      R     #tbMSTO; // Output MSTO

      U     #tbMSTA; // Output MSTA
      =     #MSTA;
      U     #tbMSTO; // Output MSTO
      =     #MSTO;

      NOP   0;
NETWORK
TITLE =Combinate States
//----Alarms----
      U     #tbCmdLock; //Command LOCK
      U(    ;
      O     #tbAuto; // AUTO!
      O     #tbManual; // MANUAL
      )     ;
      L     6; // Lock
      SPB   COD1;
      U     #tbCmdEmergOff; // Emergency Off
      L     7;
      SPB   COD1;
      UN    #tbExtFaultA; // External Fault Alarm
      UN    #tbActionA; // Action alarm
      UN    #tbNonFeedbackA; // Non -Feedback alarm
      UN    #tbAutoA; // Auto failure alarm
      UN    #tbBlackout; // Input Blackout
      L     1; // Normal
      SPB   COD1;
      U     #tbExtFaultA; // External Fault Alarm
      L     2;
      SPB   COD1;
      U     #tbAutoA; // Auto failure alarm
      L     3;
      SPB   COD1;
      U     #tbActionA; // Action alarm
      L     4;
      SPB   COD1;
      U     #tbNonFeedbackA; // Non -Feedback alarm
      L     5;
      SPB   COD1;
      U     #tbBlackout; // Input Blackout
      L     8;
      SPB   COD1;

      L     0; //Undefined
COD1: T     LW    10; //States to OS

//----Status----

      O     #BLKO; //Backout
      O     #tbBlackoutStartTact; // BLACKOUT START timer actic
      L     5; //Blackout
      SPB   COD2;
      U     #tbRunning; //Input Running
      L     1; //Running
      SPB   COD2;
      U     #tbAuto; // AUTO!
      UN    #tbStartTact; // START Timer activ
      UN    #tbExtFaultA; // External Fault Alarm
      UN    #tbActionA; // Action alarm
      UN    #tbNonFeedbackA; // Non -Feedback alarm
      UN    #tbAutoA; // Auto failure alarm
      UN    #tbBlackout; // Input Blackout
      U     #tbAutoStbyCtrl; //Standbycontrol active
      L     4; //Standby
      SPB   COD2;
      UN    #tbRunning; //Not Running
      U     #tbMSTA; // Start!
      L     3; //Starting
      SPB   COD2;
      UN    #tbRunning; //Input Stopped
      L     2; //Stopped
      SPB   COD2;
      L     0; //Undefined
COD2: T     LW    12; //States to OS

      UN    #tbRemote; //Local?
      L     256;
      SPB   COD3;
      U     #tbManual; //Manual?
      L     512;
      SPB   COD3;
      U     #tbAuto; // AUTO?
      L     1024;
      SPB   COD3;
      L     0;
COD3: L     LW    12; //Basic states
      +I    ;
      T     LW    12; //Combinate states to OS

NETWORK
TITLE =Store States in Record

      L     0; // Reset Commands OS
      T     #Motor1.CmdOS;
      T     #OSCOM; // Write Reset Back to I/O interface  added: 20060619 /Ho
      L     LW    10;
      T     #Motor1.AlarmOS; // Alarms to OS
      T     #OSALARM;
      L     LW    12;
      T     #Motor1.StatusOS; // States to OS
      T     #OSSTAT;
      L     LW    14;
      T     #Motor1.Status1; // Status stored
      L     LW    16;
      T     #Motor1.Status2; // Status stored


NETWORK
TITLE =Write record

      CALL "BLKMOV" (
           SRCBLK                   := #Motor1,
           RET_VAL                  := #siFailWR,
           DSTBLK                   := #P_currentRecord);


END_FUNCTION_BLOCK

